| TEXAS INSTRUMENTS INCORPORATED
| Standard Linear and Logic Group
| IBIS Model of SN74AC245
| OCTAL BUS TRANSCEIVERS WITH 3-STATE OUTPUTS
| This file contains package information for the following:
|  PDIP 20-pin (N) package as [Component] AC245_N
|  SSOP 20-pin (DB) package as [Component] AC245_DB
|  SOIC 20-pin (DW) package as [Component] AC245_DW
|  SOP 20-pin (NS) package as [Component] AC245_NS
|  TSSOP 20-pin (PW) package as [Component] AC245_PW
| This device can be powered at the following Vccs:
|  5 volt Vcc
|  3.3 volt Vcc
| This file provides unique models under the [Model Selector] for each Vcc.
| For operation at a specific Vcc, select the appropriate model after each
| [Model Selector] keyword.
[IBIS Ver]   3.2
[Comment char]  |_char
[File Name]   sn74ac245.ibs
[File Rev]   1.1 | a_die
[Date]   March 13, 2006
[Source]   Data created from TI-SPICE simulations at TI-SLL.
[Notes]   The following is an IBIS list for the SN74AC245.
   Please contact sllibis@ti.com with questions and
   comments concerning SLL IBIS models.
   This IBIS model is created from a BA (back annotated netlist)
   - FILE REV HISTORY
   - 1.1 Release IBIS file on 03/17/06
[Disclaimer] Property of Texas Instruments Incorporated.  Unauthorized
   reproduction and/or distribution is strictly prohibited.
   This product is protected under copyright law.
   Created  2006, (C) Copyright  2006, Texas Instruments
   Incorporated, All Rights Reserved
   UNLESS THERE IS A SIGNED, WRITTEN AGREEMENT TO THE
   CONTRARY, TEXAS INSTRUMENTS (TI) IS PROVIDING THE IBIS
   MODELS  AND WITHOUT ANY WARRANTY, EXPRESSED OR
   IMPLIED.  TI assumes no liability for:
   1) the accuracy of the IBIS models provided to your
   company;
   2) the proper functioning of these IBIS Models in your
   design or for any resulting applications; or
   3) infringement of patents, copyrights or intellectual
   property rights resulting from your use of these IBIS
   models.
   TI provides IBIS Models as a service to our customers.
   You and your company shall not distribute, sell or give
   these models to anyone else without prior written
   permission from TI.
   TI reserves the right to make changes to our products or
   to discontinue any semiconductor product or service
   without notice, and advises our customers to obtain the
   latest version of relevant information to verify, before
   placing orders, that the information being relied on is
   current.
   Please be aware that your receipt and use of the IBIS
   information provided shall serve as acceptance of these
   terms and conditions.  If you do not accept these terms,
   you should return or destroy the IBIS models and any
   other accompanying information immediately.
| Component SN74AC245_N 20-PIN PDIP
[Component]   SN74AC245_N
[Manufacturer]   Texas Instruments, Inc.
[Package]
|   typ   min   max
R_pkg   4.300e-02   3.800e-02   5.000e-02
L_pkg   7.384e-09   4.680e-09   1.032e-08
C_pkg   5.100e-13   2.310e-13   8.210e-13
[Pin]   signal_name   model_name   R_pin   L_pin   C_pin
1   DIR   AC245_DIR   4.200e-02   9.427e-09   8.100e-13
2   A1   AC245_IO   4.600e-02   8.544e-09   4.560e-13
3   A2   AC245_IO   4.800e-02   7.163e-09   4.350e-13
4   A3   AC245_IO   4.000e-02   4.825e-09   2.610e-13
5   A4   AC245_IO   4.000e-02   5.284e-09   6.480e-13
6   A5   AC245_IO   4.000e-02   4.686e-09   2.320e-13
7   A6   AC245_IO   4.000e-02   6.359e-09   4.890e-13
8   A7   AC245_IO   3.800e-02   7.982e-09   4.750e-13
9   A8   AC245_IO   4.300e-02   9.403e-09   4.750e-13
10   GND   GND   5.000e-02   1.032e-08   8.050e-13
11   B8   AC245_IO   5.000e-02   1.028e-08   8.100e-13
12   B7   AC245_IO   4.300e-02   9.383e-09   4.770e-13
13   B6   AC245_IO   3.800e-02   7.978e-09   4.760e-13
14   B5   AC245_IO   4.000e-02   6.302e-09   4.920e-13
15   B4   AC245_IO   4.000e-02   4.680e-09   2.310e-13
16   B3   AC245_IO   4.000e-02   5.284e-09   6.480e-13
17   B2   AC245_IO   4.000e-02   4.822e-09   2.610e-13
18   B1   AC245_IO   4.700e-02   7.118e-09   4.390e-13
19   NOE   AC245_NOE   4.600e-02   8.492e-09   4.610e-13
20   VCC   POWER   4.300e-02   9.348e-09   8.210e-13
| Component SN74AC245_DB 20-PIN SSOP
[Component]   SN74AC245_DB
[Manufacturer]   Texas Instruments, Inc.
[Package]
|   typ   min   max
R_pkg   4.000e-02   3.500e-02   5.100e-02
L_pkg   3.495e-09   3.035e-09   4.314e-09
C_pkg   4.200e-13   3.460e-13   5.020e-13
[Pin]   signal_name   model_name   R_pin   L_pin   C_pin
1   DIR   AC245_DIR   4.900e-02   4.310e-09   5.020e-13
2   A1   AC245_IO   4.800e-02   3.903e-09   4.870e-13
3   A2   AC245_IO   3.500e-02   3.189e-09   3.960e-13
4   A3   AC245_IO   3.500e-02   3.036e-09   3.470e-13
5   A4   AC245_IO   3.500e-02   3.035e-09   3.670e-13
6   A5   AC245_IO   3.500e-02   3.035e-09   3.670e-13
7   A6   AC245_IO   3.500e-02   3.036e-09   3.470e-13
8   A7   AC245_IO   3.500e-02   3.189e-09   3.970e-13
9   A8   AC245_IO   4.700e-02   3.899e-09   4.880e-13
10   GND   GND   5.100e-02   4.314e-09   5.000e-13
11   B8   AC245_IO   5.100e-02   4.314e-09   5.000e-13
12   B7   AC245_IO   4.700e-02   3.899e-09   4.880e-13
13   B6   AC245_IO   3.500e-02   3.189e-09   3.970e-13
14   B5   AC245_IO   3.500e-02   3.036e-09   3.460e-13
15   B4   AC245_IO   3.500e-02   3.035e-09   3.670e-13
16   B3   AC245_IO   3.500e-02   3.035e-09   3.670e-13
17   B2   AC245_IO   3.500e-02   3.036e-09   3.460e-13
18   B1   AC245_IO   3.500e-02   3.189e-09   3.970e-13
19   NOE   AC245_NOE   4.700e-02   3.899e-09   4.880e-13
20   VCC   POWER   5.100e-02   4.314e-09   5.020e-13
| Component SN74AC245_DW 20-PIN SOIC
[Component]   SN74AC245_DW
[Manufacturer]   Texas Instruments, Inc.
[Package]
|   typ   min   max
R_pkg   3.800e-02   3.300e-02   4.500e-02
L_pkg   5.012e-09   4.110e-09   6.349e-09
C_pkg   7.170e-13   5.300e-13   8.680e-13
[Pin]   signal_name   model_name   R_pin   L_pin   C_pin
1   DIR   AC245_DIR   4.200e-02   6.336e-09   8.650e-13
2   A1   AC245_IO   4.300e-02   5.542e-09   8.670e-13
3   A2   AC245_IO   3.400e-02   4.714e-09   7.320e-13
4   A3   AC245_IO   3.400e-02   4.377e-09   5.910e-13
5   A4   AC245_IO   3.600e-02   4.130e-09   5.330e-13
6   A5   AC245_IO   3.500e-02   4.111e-09   5.300e-13
7   A6   AC245_IO   3.400e-02   4.284e-09   5.830e-13
8   A7   AC245_IO   3.400e-02   4.634e-09   7.260e-13
9   A8   AC245_IO   4.000e-02   5.518e-09   8.650e-13
10   GND   GND   4.300e-02   6.349e-09   8.660e-13
11   B8   AC245_IO   4.100e-02   6.281e-09   8.610e-13
12   B7   AC245_IO   4.500e-02   5.561e-09   8.680e-13
13   B6   AC245_IO   3.300e-02   4.778e-09   7.420e-13
14   B5   AC245_IO   3.500e-02   4.414e-09   5.960e-13
15   B4   AC245_IO   3.500e-02   4.110e-09   5.330e-13
16   B3   AC245_IO   3.600e-02   4.130e-09   5.330e-13
17   B2   AC245_IO   3.400e-02   4.377e-09   5.910e-13
18   B1   AC245_IO   3.400e-02   4.714e-09   7.310e-13
19   NOE   AC245_NOE   4.300e-02   5.569e-09   8.680e-13
20   VCC   POWER   4.200e-02   6.308e-09   8.640e-13
| Component SN74AC245_NS 20-PIN SOP
[Component]   SN74AC245_NS
[Manufacturer]   Texas Instruments, Inc.
[Package]
|   typ   min   max
R_pkg   4.400e-02   2.900e-02   5.800e-02
L_pkg   3.666e-09   2.317e-09   5.115e-09
C_pkg   5.480e-13   3.160e-13   7.250e-13
[Pin]   signal_name   model_name   R_pin   L_pin   C_pin
1   DIR   AC245_DIR   5.800e-02   5.115e-09   7.250e-13
2   A1   AC245_IO   5.300e-02   4.591e-09   7.240e-13
3   A2   AC245_IO   4.900e-02   3.754e-09   5.720e-13
4   A3   AC245_IO   2.900e-02   2.549e-09   3.880e-13
5   A4   AC245_IO   3.100e-02   2.317e-09   3.160e-13
6   A5   AC245_IO   3.100e-02   2.317e-09   3.160e-13
7   A6   AC245_IO   2.900e-02   2.556e-09   3.990e-13
8   A7   AC245_IO   4.900e-02   3.754e-09   5.790e-13
9   A8   AC245_IO   5.300e-02   4.591e-09   7.240e-13
10   GND   GND   5.800e-02   5.115e-09   7.250e-13
11   B8   AC245_IO   5.800e-02   5.115e-09   7.250e-13
12   B7   AC245_IO   5.300e-02   4.591e-09   7.240e-13
13   B6   AC245_IO   4.900e-02   3.754e-09   5.790e-13
14   B5   AC245_IO   2.900e-02   2.557e-09   3.990e-13
15   B4   AC245_IO   3.100e-02   2.317e-09   3.160e-13
16   B3   AC245_IO   3.100e-02   2.317e-09   3.160e-13
17   B2   AC245_IO   2.900e-02   2.557e-09   3.990e-13
18   B1   AC245_IO   4.900e-02   3.754e-09   5.790e-13
19   NOE   AC245_NOE   5.300e-02   4.591e-09   7.240e-13
20   VCC   POWER   5.800e-02   5.115e-09   7.250e-13
| Component SN74AC245_PW 20-PIN TSSOP
[Component]   SN74AC245_PW
[Manufacturer]   Texas Instruments, Inc.
[Package]
|   typ   min   max
R_pkg   5.000e-02   4.200e-02   6.000e-02
L_pkg   2.802e-09   2.248e-09   3.553e-09
C_pkg   3.170e-13   2.020e-13   4.430e-13
[Pin]   signal_name   model_name   R_pin   L_pin   C_pin
1   DIR   AC245_DIR   5.500e-02   3.461e-09   4.400e-13
2   A1   AC245_IO   5.500e-02   3.150e-09   4.010e-13
3   A2   AC245_IO   4.200e-02   2.619e-09   3.020e-13
4   A3   AC245_IO   4.500e-02   2.273e-09   2.020e-13
5   A4   AC245_IO   4.500e-02   2.248e-09   2.240e-13
6   A5   AC245_IO   4.500e-02   2.273e-09   2.260e-13
7   A6   AC245_IO   4.400e-02   2.323e-09   2.050e-13
8   A7   AC245_IO   4.600e-02   2.704e-09   3.070e-13
9   A8   AC245_IO   6.000e-02   3.265e-09   4.110e-13
10   GND   GND   5.700e-02   3.506e-09   4.360e-13
11   B8   AC245_IO   5.800e-02   3.553e-09   4.370e-13
12   B7   AC245_IO   5.800e-02   3.193e-09   4.050e-13
13   B6   AC245_IO   4.200e-02   2.704e-09   3.110e-13
14   B5   AC245_IO   4.600e-02   2.392e-09   2.100e-13
15   B4   AC245_IO   4.700e-02   2.334e-09   2.290e-13
16   B3   AC245_IO   4.700e-02   2.300e-09   2.270e-13
17   B2   AC245_IO   4.700e-02   2.349e-09   2.070e-13
18   B1   AC245_IO   4.500e-02   2.677e-09   3.060e-13
19   NOE   AC245_NOE   6.000e-02   3.235e-09   4.060e-13
20   VCC   POWER   5.600e-02   3.487e-09   4.430e-13
| Model AC245_NOE
[Model Selector]   AC245_NOE
AC245_NOE_50   5 volt Vcc
AC245_NOE_33   3.3 volt Vcc
| Model AC245_DIR
[Model Selector]   AC245_DIR
AC245_DIR_50   5 volt Vcc
AC245_DIR_33   3.3 volt Vcc
| Model AC245_IO
[Model Selector]   AC245_IO
AC245_IO_50   5 volt Vcc
AC245_IO_33   3.3 volt Vcc
| Models and submodels in the file (6): AC245_NOE_50 (Input), AC245_NOE_33 (Input), AC245_DIR_50 (Input), AC245_DIR_33 (Input), AC245_IO_50 (I/O), AC245_IO_33 (I/O)
